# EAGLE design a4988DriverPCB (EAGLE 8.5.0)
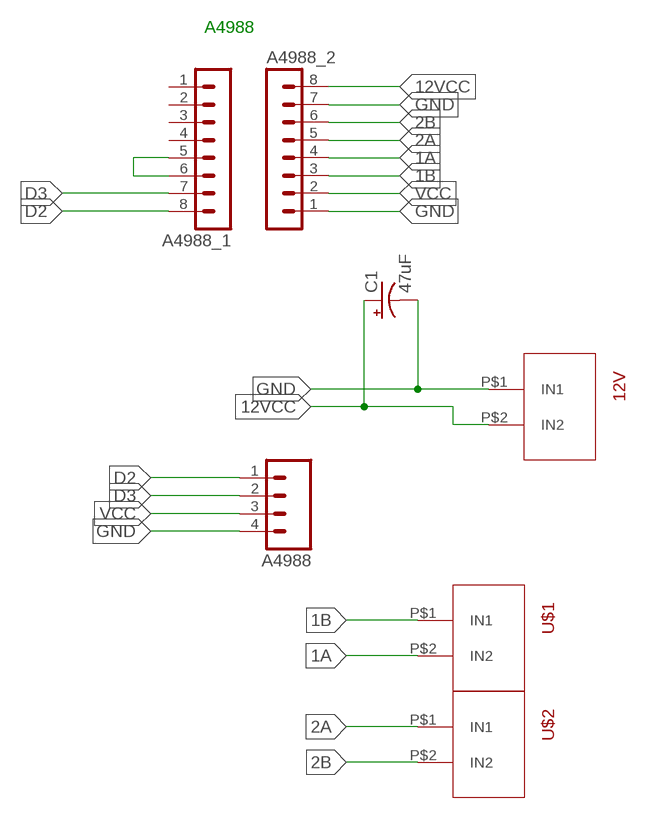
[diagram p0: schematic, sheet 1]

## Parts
12V  TERMINAL3.5MM  [TERMINALBLOCK]
A4988  M04  [04P]
A4988_1  MA08-1  [MA08-1]
A4988_2  MA08-1  [MA08-1]
C1  47uF  1000UF-RADIAL-5MM-35V-20%-KIT  [CPOL-RADIAL-5MM-10MM-KIT]
U$1  TERMINAL3.5MM  [TERMINALBLOCK]
U$2  TERMINAL3.5MM  [TERMINALBLOCK]

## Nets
1A: A4988_2.4 U$1.P$2(IN2)
1B: A4988_2.3 U$1.P$1(IN1)
2A: A4988_2.5 U$2.P$1(IN1)
2B: A4988_2.6 U$2.P$2(IN2)
12VCC: 12V.P$2(IN2) A4988_2.8 C1.+
D2: A4988.1 A4988_1.8
D3: A4988.2 A4988_1.7
GND: 12V.P$1(IN1) A4988.4 A4988_2.1 A4988_2.7 C1.-
N$1: A4988_1.5 A4988_1.6
VCC: A4988.3 A4988_2.2
Unconnected: A4988_1.1 A4988_1.2 A4988_1.3 A4988_1.4

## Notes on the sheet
- A4988

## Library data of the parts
12V U$1 U$2 = TerminalJack2pins:TERMINAL3.5MM
A4988 = con-amp-quick:M04: AMP QUICK CONNECTOR; OC_FARNELL: unknown; OC_NEWARK: unknown
A4988_1 A4988_2 = con-lstb:MA08-1: PIN HEADER; OC_FARNELL: unknown; OC_NEWARK: unknown
C1 = SparkFun-Capacitors:1000UF: 1,000µF/1mF ceramic capacitors; PROD_ID: CAP-09538; VALUE: 1mf

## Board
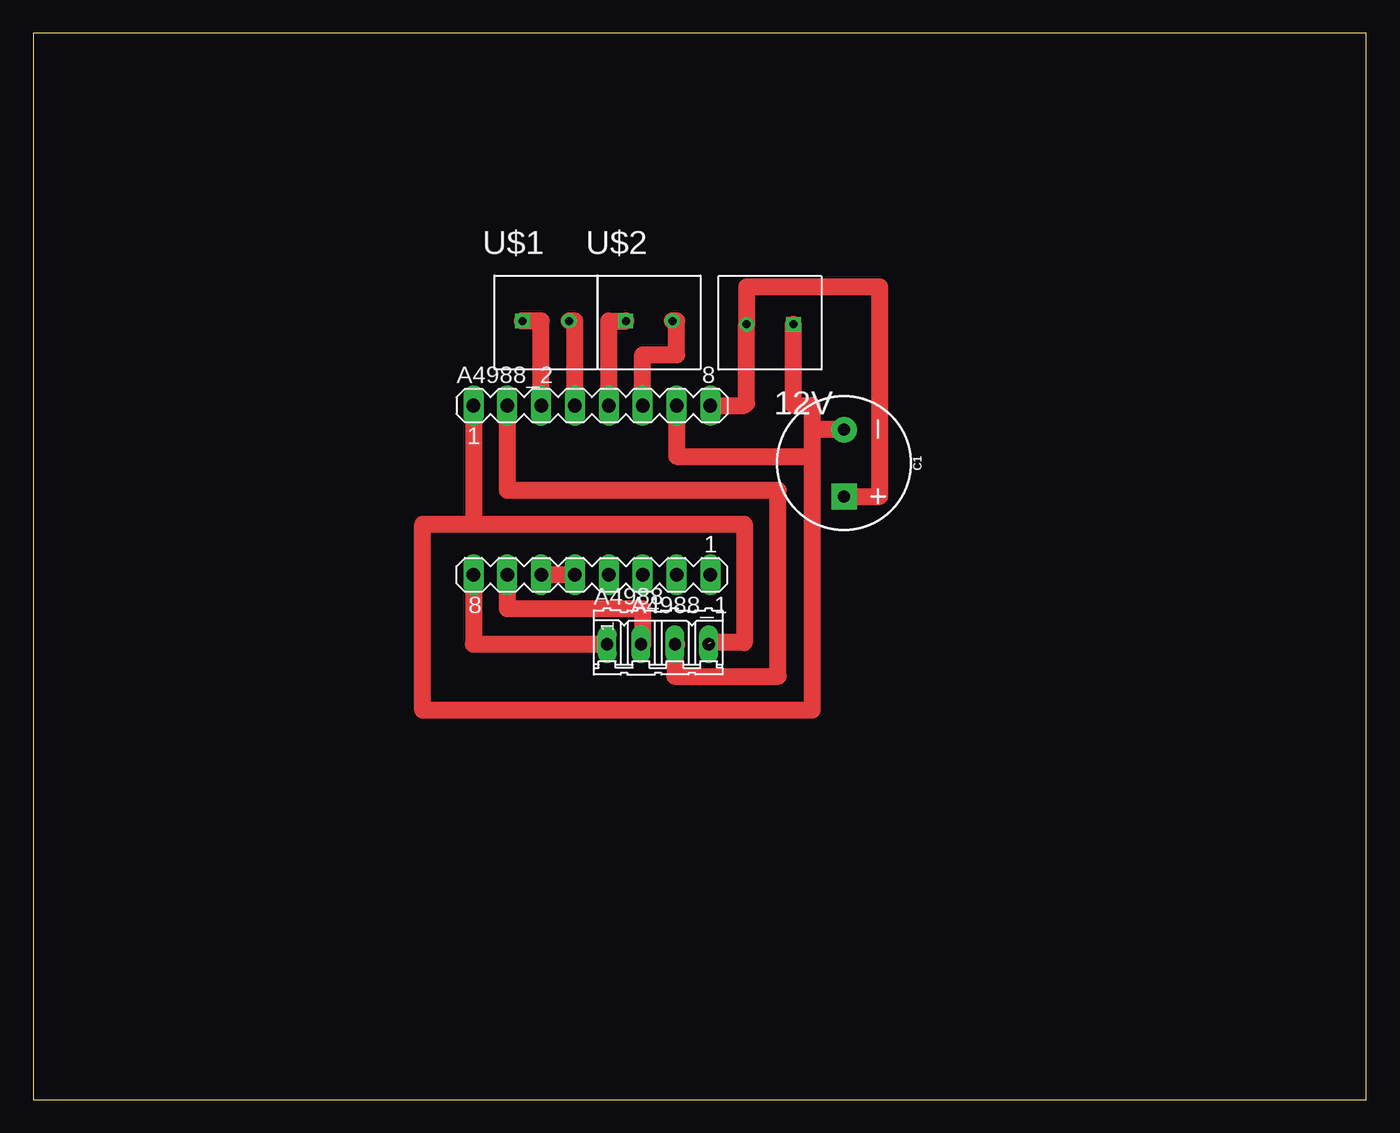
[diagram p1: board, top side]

Size 100 x 80 mm. Coordinates in mm from the lower left corner, seen from the top.
Outline: 0,0 100,0 100,80 0,80 0,0
Copper layers (1*16): Top 0.035mm / dielectric 1.5mm / Bottom 0.035mm
Design rules "default": minimum track width 6mil, minimum drill 0.35mm, track to track 6mil, track to pad 6mil, pad to pad 6mil, via to via 6mil, smd to smd 6mil, copper to edge 40mil, drill to drill 6mil, minimum pad ring 10mil, minimum via ring 8mil, stop-mask expansion 4mil, vias tented up to drill 0mil, thermal gap 10mil

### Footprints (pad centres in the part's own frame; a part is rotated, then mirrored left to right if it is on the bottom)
TERMINALBLOCK = drill 0.6 square: P$1 0,0 | drill 0.6: P$2 3.5,0
04P = drill 0.914 long: 1 -3.81,0; 2 -1.27,0; 3 1.27,0; 4 3.81,0
MA08-1 = drill 1.016 long: 1 -8.89,0; 2 -6.35,0; 3 -3.81,0; 4 -1.27,0; 5 1.27,0; 6 3.81,0; 7 6.35,0; 8 8.89,0
CPOL-RADIAL-5MM-10MM-KIT = drill 0.9 pad 1.93 square: + 2.5,0 | drill 0.9 pad 1.93: - -2.5,0

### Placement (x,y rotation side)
12V  57.02,58.17 180 top
A4988  46.86,34.16 0 top
A4988_1  41.91,39.37 180 top
A4988_2  41.91,52.07 0 top
C1  60.83,47.75 270 top
U$1  36.7,58.42 0 top
U$2  44.45,58.42 0 top

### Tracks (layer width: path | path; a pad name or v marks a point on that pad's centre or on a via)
1A
  Top 1.27: A4988_2.4 40.64,58.42 U$1.P$2
1B
  Top 1.27: A4988_2.3 38.1,58.42 U$1.P$1
2A
  Top 1.27: A4988_2.5 43.18,58.42 U$2.P$1
2B
  Top 1.27: A4988_2.6 45.72,55.88 48.26,55.88 48.26,58.42 U$2.P$2
12VCC
  Top 1.27: C1.+ 63.5,45.25 63.5,60.96 53.52,60.96 12V.P$2 53.52,52.25 53.34,52.07 A4988_2.8
D2
  Top 1.27: A4988_1.8 33.02,34.16 A4988.1
D3
  Top 1.27: A4988_1.7 35.56,36.83 45.72,36.83 45.72,34.16 A4988.2
GND  (1 unrouted)
  Top 1.27: 12V.P$1 57.02,52.07 58.42,52.07 58.42,50.25 | 33.02,43.18 29.21,43.18 29.21,29.21 58.42,29.21 58.42,48.26 | 33.02,43.18 53.34,43.18 53.34,34.29 50.8,34.29 | 58.42,50.25 58.42,48.26 | A4988_2.1 33.02,43.18 | A4988_2.7 48.26,48.26 58.42,48.26 | C1.- 58.42,50.25
N$1
  Top 1.27: A4988_1.5 A4988_1.6
VCC
  Top 1.27: 48.26,34.16 A4988.3 48.13,31.75 55.88,31.75 55.88,45.72 35.56,45.72 A4988_2.2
